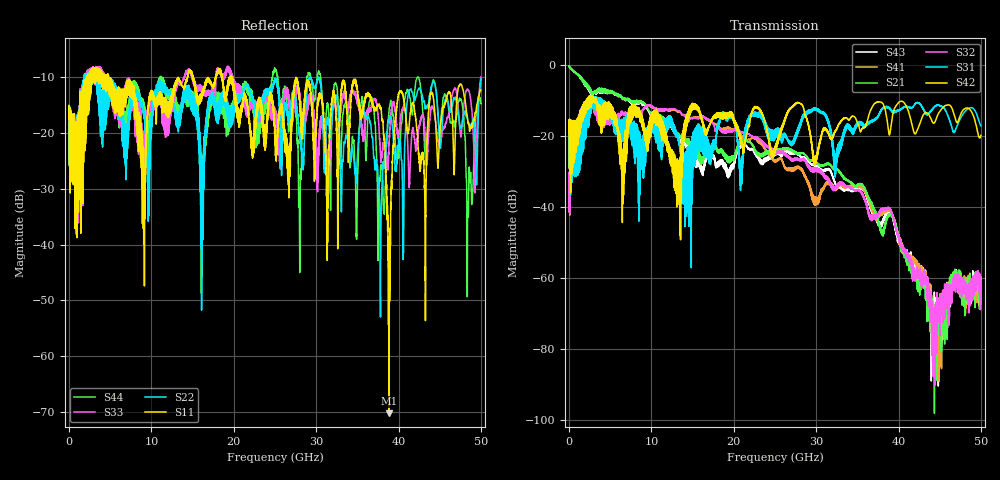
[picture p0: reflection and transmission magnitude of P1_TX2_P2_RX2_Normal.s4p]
!Keysight Technologies,N5225A,MY51441389,A.10.49.11
!Date: Monday, July 08, 2019 15:19:27
!Correction: S11(Full 4 Port(1,2,3,4))
!S12(Full 4 Port(1,2,3,4))
!S13(Full 4 Port(1,2,3,4))
!S14(Full 4 Port(1,2,3,4))
!S21(Full 4 Port(1,2,3,4))
!S22(Full 4 Port(1,2,3,4))
!S23(Full 4 Port(1,2,3,4))
!S24(Full 4 Port(1,2,3,4))
!S31(Full 4 Port(1,2,3,4))
!S32(Full 4 Port(1,2,3,4))
!S33(Full 4 Port(1,2,3,4))
!S34(Full 4 Port(1,2,3,4))
!S41(Full 4 Port(1,2,3,4))
!S42(Full 4 Port(1,2,3,4))
!S43(Full 4 Port(1,2,3,4))
!S44(Full 4 Port(1,2,3,4))
!S4P File: Measurements: <S11,S12,S13,S14>,
!<S21,S22,S23,S24>,
!<S31,S32,S33,S34>,
!<S41,S42,S43,S44>:
# Hz S  dB  R 50
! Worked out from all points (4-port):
!   5000 points, 10 MHz to 50 GHz, reference 50 ohm
!   strongest paths, dB at 10 MHz, 12.51 GHz, 25.01 GHz, 37.51 GHz, 50 GHz:
!     S42: -19.1, -26.0, -24.1, -10.4, -19.9
!     S31: -19.0, -17.7, -19.2, -14.3, -17.1
!     S32: -32.6, -12.4, -24.2, -42.9, -61.8
!     S21: -0.4, -17.2, -24.1, -43.9, -62.1
!     S41: -32.5, -12.6, -26.8, -43.3, -59.7
!     S43: -0.4, -17.9, -25.1, -45.1, -64.8
!   lowest |S11| = -70.3 dB at 38.83 GHz (marker M1), VSWR 1.00, Z = 50 - j0.0257 ohm
!   |S11| at or under -10 dB: 4.83 GHz to 13.25 GHz (8.419 GHz wide, 93.1 % of centre); 19.82 GHz to 27.57 GHz (7.75 GHz wide, 32.7 % of centre); 27.57 GHz to end of sweep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
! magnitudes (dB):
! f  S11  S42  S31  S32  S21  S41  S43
! 10 MHz  -17.5  -19.1  -19.0  -32.6  -0.4  -32.5  -0.4
! 9.68 GHz  -14.5  -18.0  -18.0  -11.3  -12.7  -11.5  -13.2
! 34.69 GHz  -10.4  -14.7  -18.4  -35.3  -34.0  -34.1  -34.8
! 38.83 GHz  -70.3  -19.4  -12.2  -40.2  -42.1  -40.6  -41.2
! 40.12 GHz  -12.6  -10.4  -12.7  -49.6  -49.4  -50.8  -49.9
! 44.62 GHz  -21.3  -15.0  -11.4  -68.7  -69.9  -79.0  -69.2
! 50 GHz  -12.3  -19.9  -17.1  -61.8  -62.1  -59.7  -64.8
